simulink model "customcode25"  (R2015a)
settings: Solver=ode3  SolverMode=SingleTasking  StartTime=0.0  StopTime=10.0  RelTol=1e-3
PreLoadFcn:
  | waijung.modelPreload; % Required for working with Waijung Blockset. Do not remove.
undefined symbols (not defined in the file): A, A4, aligned, bits, disable_customio, enable_customio, GPIO_Pin_4, HSEOSC, hseosc8mhz, In1, in1, Link, LQFP100, Out1, out1, output_customio, Raw, right, ST, start_customio, stm32f4, STM32F407VG, STM32F40_41xxx, stm32f4_io_customcode, stm32f4_target, system_stm32f4xx_default, targets, unit16, utils, waijung17_03a
libraries: waijung_customcode x1, stm32f4_adc_lib x1, stm32f4_dac_lib x1, stm32f4_device_config_lib x1

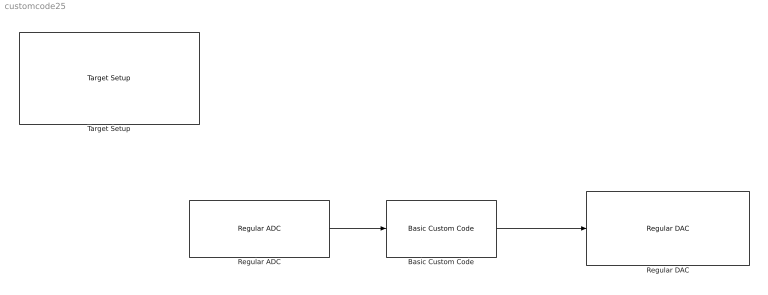
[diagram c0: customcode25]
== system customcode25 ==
  Basic Custom Code : waijung_customcode/Basic Custom Code  inputporttype=uint16_t  cinputportlabel=In1  cinputportlabelstr="[\"In1\"]"  inputportcount=1  inputporttypeid=[-1]  outputporttype=uint16_t  coutputportlabel=Out1  coutputportlabelstr="[\"Out1\"]"  outputportcount=1  outputporttypeid=[-1]  incpath={fullfile(pwd,'customcode0225')}  srcpath={fullfile(pwd,'customcode0225')}  incfiles={'stm32f4_io_customcode.h'}  srcfiles={'stm32f4_io_customcode.c'}  initialfuncallstr=start_customio();  enablefuncallstr=enable_customio();  outputfuncallstr=output_customio(in1,out1);  disablefuncallstr=disable_customio();  sampletime=0.01  sampletimestr=0.01  blockid=BasicCustomCode  enablecustomportlabel=on  incfilestrarray="[\"stm32f4_io_customcode.h\"]"  inputportdiminfo="[1  1  1 -1]"  outputportdiminfo="[1  1  1 -1]"
  Regular ADC : stm32f4_adc_lib/Regular ADC  adcmodule=1  outputdatatype=Raw (uint16)  prescaler=2  prescalerstr=ADC_Prescaler_Div2  chsamplingtime=Auto  chsamplingtimestr=ADC_SampleTime_480Cycles  read_an0=off  read_an1=off  read_an2=off  read_an3=off  read_an4=off  read_an5=on  read_an6=off  read_an7=off  read_an8=off  read_an9=off  read_an10=off  read_an11=off  read_an12=off  read_an13=off  read_an14=off  read_an15=off  read_an16=off  read_an17=off  read_an18=off  pinstr=GPIO_Pin_5  usedpinarray="[0  0  0  0  0  1  0  0  0  0  0  0  0  0  0  0  0  0  0]"  usedportidarray=[0]  usedpinidarray=[5]  usedpinidcount=1  sampletime=0.01  blockid=RegularADC  enablecustomportlabel=off  cinputportlabel=0  coutputportlabel=Out1, Out2
  Regular DAC : stm32f4_dac_lib/Regular DAC  inputtype=Raw 12 bits (unit16 right-aligned)  inputtypestr=Raw  dac1on=on  dac2on=off  advancedsettings=off  vref=3.3  dacbuffer=Enable  dacbufferstr=DAC_OutputBuffer_Enable  sampletime=0.01  blockid=RegularDAC  enablecustomportlabel=off  cinputportlabel=Signal1, Signal2  coutputportlabel=0  apb=1  portpinstr=A4,  portstr="[\"A\"]"  pinstr="[\"GPIO_Pin_4\"]"  pinmat=[1 4]  chmat=[1]  dacmode=DAC1  dacalignment=DAC_Align_12b_R  dacaddress=40007408
  Target Setup : stm32f4_device_config_lib/Target Setup  Priority=100  compiler=GNU ARM  previous_compiler=GNU ARM  mcu=STM32F407VG (LQFP100)  mcustr=STM32F407VG  clockconfig=HSEOSC-8MHz  system_stm32f4xx_c_path=E:\waijung17_03a\targets\stm32f4_target\stm32f4\utils\system_stm32f4xx_default\STM32F40_41xxx\hseosc8mhz  showmemoryconfiguration=off  stacksize=0x2000  heapsize=0x2000  enableautocompiledownload=on  fullchiperase=off  programmerinterface=ST-Link  editctrlstr=on  compilercontrolstr=$(patsubst %, -I%, .) -mcpu=cortex-m4 -mthumb -mthumb-interwork -mfloat-abi=hard -mfpu=fpv4-sp-d16 -ffast-math -Wall -Wextra -Ofast  assemblercontrolstr=$(patsubst %, -I%, .) -mcpu=cortex-m4 -mthumb -mthumb-interwork -mfloat-abi=hard -mfpu=fpv4-sp-d16 -ffast-math -Wall -Wextra -Ofast -Wa,-amhls=$(<:.s=.lst) -D__STACK_SIZE=$(STACK_SIZE) -D__HEAP_SIZE=$(HEAP_SIZE)  linkercontrolstr=-T$(LD_SCRIPT) -g -Wl,-Map=$(MAP),--cref,--no-warn-mismatch -mcpu=cortex-m4 -mthumb -mthumb-interwork -mfloat-abi=hard -mfpu=fpv4-sp-d16 -specs=nosys.specs  runafterdownload=on  execprofile=None  profileruart=3  profilerbaud=500000  profilertxpin=D8  profilerinitstr=0.01,168000000,1680000,500000,0  manualsetsampletime=off  sampletime=0.01  blockid=TargetSetup  systickreloadvalue=1680000  hseval=8000000  lastprofileruart=3  hclk=168000000  flashorigin=0x8000000  flashlength=1024k  ramorigin=0x20000000  ramlength=128k  useextram=off
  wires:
  Regular ADC/1 -> Basic Custom Code/1
  Basic Custom Code/1 -> Regular DAC/1
